|IBIS PowerSpan II Single-PCI IBIS Model for the 35 mm HSBGA Package
|MOdel is applicable to the following Tundra Part Numbers:
|CA91L8260B-100CE
[IBIS Ver]   3.2
[Comment char]  |_char
[File name]   a101am11.ibs
[File Rev]   1.1
[Date]   Feb 20, 2002
[Source]   SPICE-to-IBIS translation
|   Temperature: 25C typ, -40C max, 125C min.
[Notes]
  Revision History:
   1.0 2/20/02 Initial release
   1.1 9/08/2009 Updated with IDT formatting
[Disclaimer] This model is subject to change.
   Integrated Device Technology, Inc. ("IDT") hereby grants the
   user of this IBIS model a non-exclusive, nontransferable
   license to use this IBIS model under the following terms. The
   user is granted this license only to use the IBIS model and is
   not granted rights to sell, copy (except as needed to run the
   IBIS model), rent, lease or sub-license the IBIS model in
   whole or in part, or in modified form to anyone. The User may
   modify the IBIS model to suit its specific applications, but
   rights to derivative works and such modifications shall belong
   to IDT. This IBIS model is provided on an AS IS" basis and IDT
   makes absolutely no warranty with respect to the information
   contained herein. IDT DISCLAIMS AND CUSTOMER WAIVES ALL
   WARRANTIES, EXPRESS AND IMPLIED, INCLUDING WARRANTIES OF
   MERCHANTABILITY AND FITNESS FOR A PARTICULAR PURPOSE. THE
   ENTIRE RISK AS TO QUALITY AND PERFORMANCE IS WITH THE USER
   ACCORDINGLY, IN NO EVENT SHALL IDT BE LIABLE FOR ANY DIRECT OR
   INDIRECT DAMAGES, WHETHER IN CONTRACT OR TORT, INCLUDING ANY
   LOST PROFITS OR OTHER INCIDENTAL, CONSEQUENTIAL, EXEMPLARY, OR
   PUNITIVE DAMAGES ARISING OUT OF THE USE OR APPLICATION OF THE
   IBIS model. Further, IDT reserves the right to make changes
   without notice to any product herein to improve reliability,
   function, or design. IDT does not convey any license under
   patent rights or any other intellectual property rights,
   including those of third parties. IDT is not obligated to
   provide maintenance or support for the licensed IBIS model.
[Copyright]   Copyright 2009, Integrated Device Technology, Inc. all
   rights reserved.
|   COMPONENT: PowerSpan II 2-Port (Single PCI)
[Component]   PowerSpan
[Manufacturer]  Integrated Device Technology, Inc.
[Package]
|variable   typ   min   max
R_pkg   161.209m   92.000m   292.000m
L_pkg   4.895n   2.790n   8.870n
C_pkg   1.795p   0.818p   2.839p
|Package parameters for Lead including bondwire inductance
[Pin] signal_name   model_name   R_pin L_pin C_pin
B21	ENUM_b		BPCIXT	178m	5.4n	1.817p
E4	ES			BLVTTL35	151m	4.58n	1.96p
J1	HEALTHY_b		BLVTTL35	172m	5.22n	1.564p
N1	I2C_SCLK		BLVTTL35	159m	4.83n	1.457p
AF9	I2C_SDA		BLVTTL35	188m	5.7n	1.698p
AF18	INT[0]_b		BLVTTL35	187m	5.68n	1.688p
AF3	INT[1]_b		BLVTTL35	249m	7.57n	2.262p
AE3	INT[2]_b		BLVTTL35	232m	7.06n	2.334p
AD1	INT[3]_b		BLVTTL35	239m	7.25n	2.117p
J4	INT[4]_b		BLVTTL35	110m	3.33n	1.614p
AB1	INT[5]_b		BLVTTL35	225m	6.82n	1.999p
A5	JT_TCK		BLVTTL35	221m	6.7n	1.964p
A3	JT_TDI		BLVTTL35	232m	7.03n	2.054p
A4	JT_TDO		BLVTTL35	231m	7.02n	2.055p
D7	JT_TMS		BLVTTL35	127m	3.86n	1.766p
AC1	JT_TRST_b		BLVTTL35	232m	7.04n	2.059p
AC7	LED_b			BLVTTL35	148m	4.51n	2.063p
B24	P1_64EN_b		BPCIXT	255m	7.76n	2.659p
F23	P1_ACK64_b		BPCIXT	159m	4.82n	2.028p
F24	P1_AD[0]		BPCIXT	179m	5.42n	2.026p
G24	P1_AD[1]		BPCIXT	165m	5n	2.097p
K25	P1_AD[10]		BPCIXT	177m	5.38n	1.792p
K24	P1_AD[11]		BPCIXT	144m	4.38n	1.857p
K23	P1_AD[12]		BPCIXT	120m	3.66n	1.697p
K26	P1_AD[13]		BPCIXT	194m	5.89n	1.744p
M24	P1_AD[14]		BPCIXT	139m	4.21n	1.675p
M23	P1_AD[15]		BPCIXT	106m	3.21n	1.605p
R26	P1_AD[16]		BPCIXT	195m	5.92n	1.77p
P23	P1_AD[17]		BPCIXT	114m	3.45n	1.7p
P24	P1_AD[18]		BPCIXT	145m	4.41n	1.767p
P25	P1_AD[19]		BPCIXT	166m	5.05n	1.723p
M26	P1_AD[2]		BPCIXT	187m	5.69n	1.697p
T25	P1_AD[20]		BPCIXT	162m	4.9n	1.671p
R24	P1_AD[21]		BPCIXT	143m	4.35n	1.713p
R25	P1_AD[22]		BPCIXT	168m	5.09n	1.754p
U24	P1_AD[23]		BPCIXT	148m	4.49n	1.772p
T23	P1_AD[24]		BPCIXT	126m	3.83n	1.742p
U25	P1_AD[25]		BPCIXT	171m	5.2n	1.791p
V24	P1_AD[26]		BPCIXT	147m	4.45n	1.737p
V23	P1_AD[27]		BPCIXT	123m	3.72n	1.796p
W25	P1_AD[28]		BPCIXT	173m	5.25n	1.803p
W24	P1_AD[29]		BPCIXT	152m	4.63n	1.812p
G26	P1_AD[3]		BPCIXT	212m	6.44n	1.892p
W23	P1_AD[30]		BPCIXT	129m	3.92n	1.827p
AC26	P1_AD[31]		BPCIXT	236m	7.18n	2.218p
B12	P1_AD[32]		BPCIXT	145m	4.41n	1.546p
B11	P1_AD[33]		BPCIXT	146m	4.44n	1.56p
A12	P1_AD[34]		BPCIXT	170m	5.15n	1.545p
D12	P1_AD[35]		BPCIXT	96m	2.92n	1.523p
D25	P1_AD[36]		BPCIXT	224m	6.81n	2.228p
C12	P1_AD[37]		BPCIXT	118m	3.57n	1.52p
E24	P1_AD[38]		BPCIXT	193m	5.86n	2.207p
B13	P1_AD[39]		BPCIXT	140m	4.25n	1.521p
G25	P1_AD[4]		BPCIXT	189m	5.74n	1.907p
A13	P1_AD[40]		BPCIXT	165m	5n	1.501p
B14	P1_AD[41]		BPCIXT	144m	4.38n	1.536p
D24	P1_AD[42]		BPCIXT	210m	6.37n	2.322p
D13	P1_AD[43]		BPCIXT	94m	2.85n	1.482p
A14	P1_AD[44]		BPCIXT	167m	5.08n	1.523p
D14	P1_AD[45]		BPCIXT	96m	2.93n	1.49p
C23	P1_AD[46]		BPCIXT	235m	7.14n	2.646p
A15	P1_AD[47]		BPCIXT	160m	4.87n	1.466p
B15	P1_AD[48]		BPCIXT	138m	4.2n	1.5p
B16	P1_AD[49]		BPCIXT	141m	4.29n	1.519p
M25	P1_AD[5]		BPCIXT	164m	4.98n	1.691p
A17	P1_AD[50]		BPCIXT	168m	5.09n	1.526p
A18	P1_AD[51]		BPCIXT	174m	5.28n	1.579p
B17	P1_AD[52]		BPCIXT	146m	4.43n	1.536p
C16	P1_AD[53]		BPCIXT	120m	3.64n	1.526p
D16	P1_AD[54]		BPCIXT	98m	2.99n	1.542p
E25	P1_AD[55]		BPCIXT	218m	6.62n	2.158p
B19	P1_AD[56]		BPCIXT	161m	4.9n	1.687p
C17	P1_AD[57]		BPCIXT	125m	3.81n	1.551p
D17	P1_AD[58]		BPCIXT	104m	3.16n	1.589p
A20	P1_AD[59]		BPCIXT	189m	5.75n	1.705p
G23	P1_AD[6]		BPCIXT	146m	4.45n	1.938p
C18	P1_AD[60]		BPCIXT	132m	4.02n	1.627p
C19	P1_AD[61]		BPCIXT	140m	4.26n	1.695p
E23	P1_AD[62]		BPCIXT	175m	5.3n	2.206p
D18	P1_AD[63]		BPCIXT	111m	3.38n	1.651p
J24	P1_AD[7]		BPCIXT	155m	4.72n	1.833p
H23	P1_AD[8]		BPCIXT	134m	4.05n	1.822p
H24	P1_AD[9]		BPCIXT	155m	4.69n	1.803p
D23	P1_AVSS		GND		187m	5.67n	2.267p
J23	P1_CBE[0]_b		BPCIXT	124m	3.77n	1.752p
L25	P1_CBE[1]_b		BPCIXT	174m	5.28n	1.777p
N24	P1_CBE[2]_b		BPCIXT	139m	4.21n	1.682p
T24	P1_CBE[3]_b		BPCIXT	139m	4.23n	1.689p
D20	P1_CBE[4]_b		BPCIXT	129m	3.92n	1.851p
C21	P1_CBE[5]_b		BPCIXT	159m	4.82n	1.897p
C20	P1_CBE[6]_b		BPCIXT	150m	4.55n	1.794p
A23	P1_CBE[7]_b		BPCIXT	220m	6.67n	1.954p
A25	P1_CLK		BPCIXT	292m	8.87n	2.62p
Y24	P1_DEVSEL_b		BPCIXT	159m	4.82n	1.863p
K22	P1_DVDD		POWER		99m	3.02n	1.815p
E22	P1_DVSS		GND		143m	4.36n	2.206p
N23	P1_FRAME_b		BPCIXT	109m	3.3n	1.611p
B23	P1_GNT[1]_b		BPCIXT	202m	6.14n	2.839p
D22	P1_GNT[2]_b		BPCIXT	161m	4.89n	2.227p
A24	P1_GNT[3]_b		BPCIXT	233m	7.07n	2.064p
J25	P1_GNT[4]_b		BPCIXT	179m	5.45n	1.824p
B20	P1_IDSEL		BPCIXT	169m	5.14n	1.752p
L23	P1_INTA_b		BPCIXT	111m	3.36n	1.633p
P26	P1_IRDY_b		BPCIXT	191m	5.81n	1.721p
D15	P1_M66EN		BPCIXT	99m	3n	0.818p
L24	P1_PAR		BPCIXT	142m	4.31n	1.701p
D19	P1_PAR64		BPCIXT	120m	3.65n	1.724p
N25	P1_PERR_b		BPCIXT	163m	4.94n	1.677p
C22	P1_REQ[1]_b		BPCIXT	170m	5.17n	1.978p
D26	P1_REQ[2]_b		BPCIXT	245m	7.43n	2.174p
B18	P1_REQ[3]_b		BPCIXT	153m	4.64n	1.618p
A19	P1_REQ[4]_b		BPCIXT	182m	5.52n	1.641p
F25	P1_REQ64_b		BPCIXT	203m	6.15n	2.027p
AC25	P1_RST_b		BPCIXT	224m	6.79n	2.324p
A8	P1_RST_DIR		BLVTTL35	190m	5.78n	1.713p
C15	P1_SERR_b		BPCIXT	123m	3.72n	1.553p
N26	P1_STOP_b		BPCIXT	187m	5.69n	1.689p
R23	P1_TEST1		BLVTTL35	116m	3.51n	1.689p
H26	P1_TEST2		BLVTTL35	212m	6.44n	1.893p
Y25	P1_TRDY_b		BPCIXT	181m	5.5n	1.866p
A22	P1_VDDA		POWER		203m	6.16n	1.906p
AD16	P2_TEST1		BLVTTL35	131m	3.97n	1.632p
J3	PB_A[0]		BLVTTL35	131m	3.97n	1.685p
G2	PB_A[1]		BLVTTL35	169m	5.12n	1.745p
C2	PB_A[10]		BLVTTL35	213m	6.48n	1.763p
D2	PB_A[11]		BLVTTL35	198m	6.03n	2.022p
D5	PB_A[12]		BLVTTL35	152m	4.62n	1.978p
B3	PB_A[13]		BLVTTL35	212m	6.44n	2.108p
D6	PB_A[14]		BLVTTL35	139m	4.21n	1.877p
C5	PB_A[15]		BLVTTL35	173m	5.25n	1.958p
C6	PB_A[16]		BLVTTL35	166m	5.05n	1.905p
C4	PB_A[17]		BLVTTL35	182m	5.53n	2.03p
B6	PB_A[18]		BLVTTL35	188m	5.7n	1.916p
B4	PB_A[19]		BLVTTL35	204m	6.2n	2.05p
H4	PB_A[2]		BLVTTL35	118m	3.57n	1.693p
B5	PB_A[20]		BLVTTL35	197m	5.99n	1.985p
B7	PB_A[21]		BLVTTL35	177m	5.38n	1.832p
C7	PB_A[22]		BLVTTL35	154m	4.67n	1.795p
D8	PB_A[23]		BLVTTL35	118m	3.6n	1.693p
D9	PB_A[24]		BLVTTL35	111m	3.37n	1.654p
C8	PB_A[25]		BLVTTL35	144m	4.38n	1.727p
B8	PB_A[26]		BLVTTL35	170m	5.17n	1.759p
C10	PB_A[27]		BLVTTL35	128m	3.89n	1.585p
D10	PB_A[28]		BLVTTL35	104m	3.15n	1.592p
C9	PB_A[29]		BLVTTL35	138m	4.18n	1.694p
G4	PB_A[3]		BLVTTL35	134m	4.05n	1.82p
A7	PB_A[30]		BLVTTL35	196m	5.95n	1.761p
D11	PB_A[31]		BLVTTL35	99m	3n	1.541p
H3	PB_A[4]		BLVTTL35	139m	4.23n	1.679p
G3	PB_A[5]		BLVTTL35	149m	4.51n	1.753p
F4	PB_A[6]		BLVTTL35	145m	4.4n	1.951p
D3	PB_A[7]		BLVTTL35	184m	5.58n	2.026p
D1	PB_A[8]		BLVTTL35	226m	6.86n	2.01p
E3	PB_A[9]		BLVTTL35	177m	5.36n	2.078p
K1	PB_AACK_b		BLVTTL35	168m	5.11n	1.533p
AF8	PB_ABB_b		BLVTTL35	200m	6.06n	1.792p
P4	PB_AP[0]		BLVTTL35	93m	2.83n	1.495p
P1	PB_AP[1]		BLVTTL35	156m	4.75n	1.452p
N4	PB_AP[2]		BLVTTL35	92m	2.79n	1.467p
N3	PB_AP[3]		BLVTTL35	114m	3.46n	1.475p
L2	PB_ARTRY_b		BLVTTL35	138m	4.2n	1.48p
AC4	PB_AVSS		GND		176m	5.34n	2.246p
L4	PB_BG1_b		BLVTTL35	97m	2.95n	1.506p
AF2	PB_BG2_b		BLVTTL35	262m	7.95n	2.364p
V1	PB_BG3_b		BLVTTL35	179m	5.43n	1.621p
B10	PB_BR1_b		BLVTTL35	151m	4.57n	1.603p
F2	PB_BR2_b		BLVTTL35	186m	5.63n	1.906p
H1	PB_BR3_b		BLVTTL35	182m	5.52n	1.645p
C25	PB_CI_b		BLVTTL35	241m	7.31n	2.354p
AF5	PB_CLK		BLVTTL35	216m	6.56n	2.014p
AD21	PB_D[0]		BLVTTL35	160m	4.86n	1.89p
AC14	PB_D[1]		BLVTTL35	105m	3.18n	1.578p
AE11	PB_D[10]		BLVTTL35	157m	4.75n	1.651p
AD7	PB_D[11]		BLVTTL35	165m	5.01n	1.979p
AA4	PB_D[12]		BLVTTL35	143m	4.34n	1.914p
Y4	PB_D[13]		BLVTTL35	133m	4.03n	1.81p
AD6	PB_D[14]		BLVTTL35	183m	5.56n	2.128p
AE7	PB_D[15]		BLVTTL35	181m	5.48n	1.84p
AF17	PB_D[16]		BLVTTL35	170m	5.16n	1.563p
AE14	PB_D[17]		BLVTTL35	155m	4.7n	1.641p
AC11	PB_D[18]		BLVTTL35	108m	3.29n	1.673p
AC9	PB_D[19]		BLVTTL35	119m	3.62n	1.758p
AD12	PB_D[2]		BLVTTL35	127m	3.85n	1.567p
Y2	PB_D[20]		BLVTTL35	183m	5.57n	1.857p
U4	PB_D[21]		BLVTTL35	109m	3.3n	1.616p
R3	PB_D[22]		BLVTTL35	116m	3.52n	1.501p
T4	PB_D[23]		BLVTTL35	106m	3.22n	1.606p
AC16	PB_D[24]		BLVTTL35	106m	3.2n	1.582p
AF14	PB_D[25]		BLVTTL35	179m	5.43n	1.62p
AF10	PB_D[26]		BLVTTL35	183m	5.55n	1.655p
AC10	PB_D[27]		BLVTTL35	119m	3.62n	1.7p
AA3	PB_D[28]		BLVTTL35	169m	5.13n	1.947p
V3	PB_D[29]		BLVTTL35	139m	4.22n	1.733p
AC6	PB_D[3]		BLVTTL35	158m	4.81n	2.015p
U1	PB_D[30]		BLVTTL35	171m	5.18n	1.554p
AD4	PB_D[31]		BLVTTL35	200m	6.08n	2.364p
AE21	PB_D[32]		BLVTTL35	178m	5.42n	1.84p
AD13	PB_D[33]		BLVTTL35	124m	3.77n	1.55p
AD11	PB_D[34]		BLVTTL35	132m	4n	1.634p
AB4	PB_D[35]		BLVTTL35	157m	4.76n	2.024p
AA2	PB_D[36]		BLVTTL35	193m	5.86n	1.957p
AD2	PB_D[37]		BLVTTL35	224m	6.8n	2.207p
AD5	PB_D[38]		BLVTTL35	187m	5.69n	2.46p
AE4	PB_D[39]		BLVTTL35	219m	6.65n	2.225p
AF20	PB_D[4]		BLVTTL35	189m	5.75n	1.707p
AE16	PB_D[40]		BLVTTL35	151m	4.59n	1.61p
AC13	PB_D[41]		BLVTTL35	104m	3.15n	1.57p
AD9	PB_D[42]		BLVTTL35	142m	4.31n	1.754p
AB3	PB_D[43]		BLVTTL35	176m	5.34n	1.983p
AB2	PB_D[44]		BLVTTL35	203m	6.16n	2.033p
W3	PB_D[45]		BLVTTL35	151m	4.57n	1.898p
U3	PB_D[46]		BLVTTL35	131m	3.97n	1.677p
R2	PB_D[47]		BLVTTL35	137m	4.17n	1.478p
AD15	PB_D[48]		BLVTTL35	132m	4n	1.65p
AF12	PB_D[49]		BLVTTL35	173m	5.24n	1.569p
V4	PB_D[5]		BLVTTL35	120m	3.64n	1.719p
AD10	PB_D[50]		BLVTTL35	136m	4.14n	1.654p
AD8	PB_D[51]		BLVTTL35	149m	4.53n	1.797p
Y1	PB_D[52]		BLVTTL35	201m	6.11n	1.806p
AC2	PB_D[53]		BLVTTL35	210m	6.39n	2.09p
U2	PB_D[54]		BLVTTL35	150m	4.57n	1.585p
T3	PB_D[55]		BLVTTL35	124m	3.76n	1.544p
AE15	PB_D[56]		BLVTTL35	152m	4.62n	1.628p
AC12	PB_D[57]		BLVTTL35	107m	3.24n	1.594p
AE10	PB_D[58]		BLVTTL35	159m	4.83n	1.656p
AE8	PB_D[59]		BLVTTL35	172m	5.23n	1.782p
T2	PB_D[6]		BLVTTL35	144m	4.38n	1.531p
W4	PB_D[60]		BLVTTL35	124m	3.77n	1.736p
AF4	PB_D[61]		BLVTTL35	237m	7.19n	2.158p
W1	PB_D[62]		BLVTTL35	191m	5.81n	1.724p
AC19	PB_D[63]		BLVTTL35	118m	3.57n	1.76p
R4	PB_D[7]		BLVTTL35	94m	2.84n	1.514p
AC22	PB_D[8]		BLVTTL35	155m	4.71n	1.993p
AD14	PB_D[9]		BLVTTL35	133m	4.03n	1.653p
AE5	PB_DBB_b		BLVTTL35	211m	6.42n	2.162p
A10	PB_DBG1_b		BLVTTL35	176m	5.33n	1.592p
B9	PB_DBG2_b		BLVTTL35	164m	4.97n	1.703p
E1	PB_DBG3_b		BLVTTL35	216m	6.54n	1.925p
AE20	PB_DP[0]		BLVTTL35	168m	5.09n	1.748p
AD20	PB_DP[1]		BLVTTL35	150m	4.54n	1.779p
AD18	PB_DP[2]		BLVTTL35	132m	4.01n	1.642p
AC18	PB_DP[3]		BLVTTL35	113m	3.42n	1.698p
AD19	PB_DP[4]		BLVTTL35	142m	4.3n	1.71p
AC20	PB_DP[5]		BLVTTL35	127m	3.85n	1.858p
AC17	PB_DP[6]		BLVTTL35	110m	3.34n	1.68p
AD17	PB_DP[7]		BLVTTL35	127m	3.87n	1.611p
AF7	PB_DVAL_b		BLVTTL35	202m	6.12n	1.808p
AB10	PB_DVDD		POWER		107m	3.25n	1.856p
AD3	PB_DVSS		GND		208m	6.32n	2.291p
AC15	PB_FAST		BLVTTL35	104m	3.15n	1.564p
C11	PB_GBL_b		BLVTTL35	125m	3.8n	1.56p
AF15	PB_RST_b		BLVTTL35	176m	5.36n	1.601p
C1	PB_RST_DIR		BLVTTL35	231m	7.01n	2.065p
AE13	PB_RSTCONF_b	BLVTTL35	152m	4.61n	1.591p
P3	PB_TA_b		BLVTTL35	113m	3.44n	1.459p
M3	PB_TBST_b		BLVTTL35	114m	3.46n	1.502p
AC3	PB_TEA_b		BLVTTL35	192m	5.82n	2.121p
Y3	PB_TEST1		BLVTTL35	161m	4.89n	1.918p
W2	PB_TEST2		BLVTTL35	172m	5.21n	1.788p
M1	PB_TS_b		BLVTTL35	158m	4.8n	1.45p
N2	PB_TSIZ[0]		BLVTTL35	135m	4.11n	1.469p
M2	PB_TSIZ[1]		BLVTTL35	135m	4.11n	1.485p
M4	PB_TSIZ[2]		BLVTTL35	93m	2.82n	1.475p
L3	PB_TSIZ[3]		BLVTTL35	117m	3.57n	1.501p
K3	PB_TT[0]		BLVTTL35	122m	3.71n	1.548p
K4	PB_TT[1]		BLVTTL35	102m	3.1n	1.584p
H2	PB_TT[2]		BLVTTL35	158m	4.79n	1.677p
G1	PB_TT[3]		BLVTTL35	191m	5.8n	1.733p
K2	PB_TT[4]		BLVTTL35	146m	4.44n	1.556p
AE9	PB_VDDA		POWER		173m	5.24n	1.863p
H25	PCI_GNT[5]_b	BPCIXT	189m	5.75n	1.896p
J26	PCI_GNT[6]_b	BPCIXT	196m	5.97n	1.764p
AB23	PCI_GNT[7]_b	BPCIXT	174m	5.28n	2.311p
C26	PCI_REQ[5]_b	BPCIXT	250m	7.6n	2.211p
E26	PCI_REQ[6]_b	BPCIXT	235m	7.13n	2.081p
W26	PCI_REQ[7]_b	BPCIXT	189m	5.74n	1.703p
AF13	PO_RST_b		BLVTTL35	174m	5.29n	1.592p
B1	TE			BLVTTL35	262m	7.96n	2.31p
| Models and submodels in the file (2): BPCIXT (I/O), BLVTTL35 (I/O)
